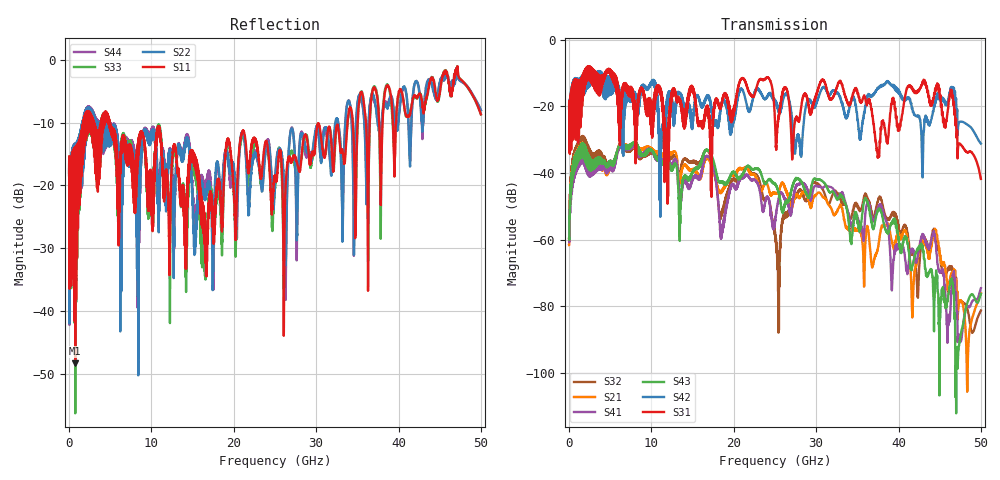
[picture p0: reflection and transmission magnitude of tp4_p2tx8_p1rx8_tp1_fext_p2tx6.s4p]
! 100G CR Analysis
! File: tp4_p2tx8_p1rx8_tp1_fext_p2tx6
! Description: 2m Cu Cable, OSFP, TP1-TP4
! Port Mapping
! Port1 -- P1RX8N
! Port2 -- P2TX6N
! Port3 -- P1RX8P
! Port4 -- P2TX6P
# GHz S MA R 50.00
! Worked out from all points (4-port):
!   5000 points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, 10 MHz to 50 GHz, reference 50 ohm
!   strongest paths, dB at 10 MHz, 12.51 GHz, 25.01 GHz, 37.51 GHz, 50 GHz:
!     S31: -20.7, -15.3, -24.9, -34.8, -41.8
!     S42: -20.5, -17.9, -18.0, -14.7, -31.2
!     S43: -59.6, -39.2, -43.2, -51.4, -76.2
!     S41: -60.2, -37.6, -54.0, -50.5, -74.6
!     S21: -61.6, -34.0, -46.3, -62.5, -76.1
!     S32: -59.8, -35.3, -57.7, -48.4, -81.3
!   lowest |S11| = -48.3 dB at 750 MHz (marker M1), VSWR 1.01, Z = 50.4 - j0.0378 ohm
!   |S11| at or under -10 dB: start of sweep to 1.719 GHz; 3.024 GHz to 3.859 GHz (834.8 MHz wide, 24.3 % of centre); 4.981 GHz to 33.81 GHz (28.83 GHz wide, 149 % of centre)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
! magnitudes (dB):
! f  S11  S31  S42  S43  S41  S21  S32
! 10 MHz  -17.9  -20.7  -20.5  -59.6  -60.2  -61.6  -59.8
! 750 MHz  -48.3  -23.9  -19.2  -36.0  -37.8  -35.8  -33.9
! 21.72 GHz  -17.8  -15.1  -20.8  -37.8  -40.7  -38.8  -38.4
! 25.4 GHz  -16.2  -23.5  -20.5  -45.6  -48.3  -45.9  -68.6
! 37.48 GHz  -6.8  -35.4  -14.6  -51.5  -50.7  -62.7  -48.6
! 43.08 GHz  -7.6  -12.9  -27.3  -65.8  -59.7  -61.2  -59.9
! 50 GHz  -8.7  -41.8  -31.2  -76.2  -74.6  -76.1  -81.3
